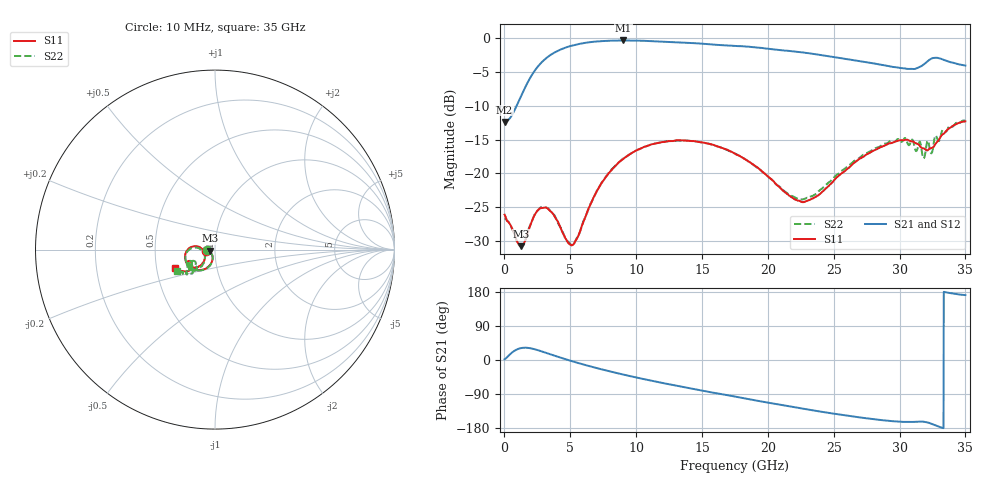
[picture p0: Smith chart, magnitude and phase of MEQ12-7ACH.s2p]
! MARKI MICROWAVE INC.
! Email:  support@markimicrowave.com  Phone:  408-778-4200
! Model Number:  MEQ12-7ACH  Date:  6/18
! Filename:		MEQ12-7ACH.S2P  Version: 1.0
! Description:  2-port S-parameter data for chip equalizer
! Features:		Low Insertion Loss, Excellent Return Loss
! Frequency Measured: 	10 MHz to 35 GHz
!S2P File: Measurements: S11, S21, S12, S22:
# Hz S  dB  R 50
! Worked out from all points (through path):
!   1601 points, 10 MHz to 35 GHz, reference 50 ohm
!   highest |S21| = -0.34 dB at 9.02 GHz (marker M1); lowest = -12.4 dB at 10 MHz (marker M2)
!   group delay of S21, straight-line fit = 17.7 ps
!   lowest |S11| = -30.8 dB at 1.257 GHz (marker M3), VSWR 1.06, Z = 47.3 - j0.587 ohm
!   |S11| at or under -10 dB: start of sweep to end of sweep
!   |S22| runs from -30.8 to -12.2 dB; largest |S21 - S12| = 0.01
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1e7  -26.12 -174.2  -12.40 2.0  -12.35 2.7  -26.66 -175.9
5.129812e8  -27.85 172.4  -11.57 17.9  -11.55 18.0  -27.97 173.1
1.256519e9  -30.78 -167.6  -8.60 31.4  -8.59 31.5  -30.73 -167.2
2.306219e9  -26.10 -148.1  -4.79 28.3  -4.79 28.3  -26.03 -147.5
2.831069e9  -25.14 -156.6  -3.56 22.7  -3.56 22.7  -24.96 -155.8
3.662081e9  -25.94 -167.6  -2.28 13.0  -2.28 13.0  -25.95 -167.8
4.996075e9  -30.53 -144.7  -1.17 -1.8  -1.17 -1.8  -30.47 -143.1
5.302238e9  -30.32 -129.5  -1.02 -4.9  -1.01 -4.9  -30.33 -130.2
5.848956e9  -27.94 -110.8  -0.79 -10.5  -0.79 -10.4  -28.00 -110.7
7.292294e9  -21.67 -106.2  -0.45 -23.9  -0.44 -23.9  -21.72 -105.3
9.019925e9  -17.87 -120.0  -0.34 -38.4  -0.35 -38.4  -17.79 -119.0
1.168791e10  -15.51 -143.9  -0.49 -58.5  -0.48 -58.4  -15.49 -141.9
1.450898e10  -15.27 -165.8  -0.75 -77.5  -0.76 -77.4  -15.29 -163.5
1.7505e10  -17.10 175.6  -1.14 -96.5  -1.15 -96.6  -17.10 178.9
2.168193e10  -23.36 -178.3  -1.91 -122.5  -1.93 -122.7  -23.22 -172.7
2.334396e10  -23.75 -150.5  -2.31 -132.4  -2.30 -132.2  -23.39 -146.1
2.686482e10  -18.00 -133.7  -3.37 -151.0  -3.39 -150.9  -17.86 -129.9
2.918291e10  -15.59 -143.0  -4.14 -160.4  -4.07 -160.6  -15.39 -140.1
3.093241e10  -15.26 -154.3  -4.55 -163.5  -4.58 -163.8  -15.04 -151.8
3.182903e10  -16.30 -153.9  -3.90 -162.9  -3.93 -162.6  -17.81 -147.4
3.287873e10  -15.30 -141.6  -2.92 -174.8  -2.86 -174.5  -14.96 -133.6
3.5e10  -12.31 -155.4  -4.05 171.2  -3.99 170.5  -12.28 -150.9
